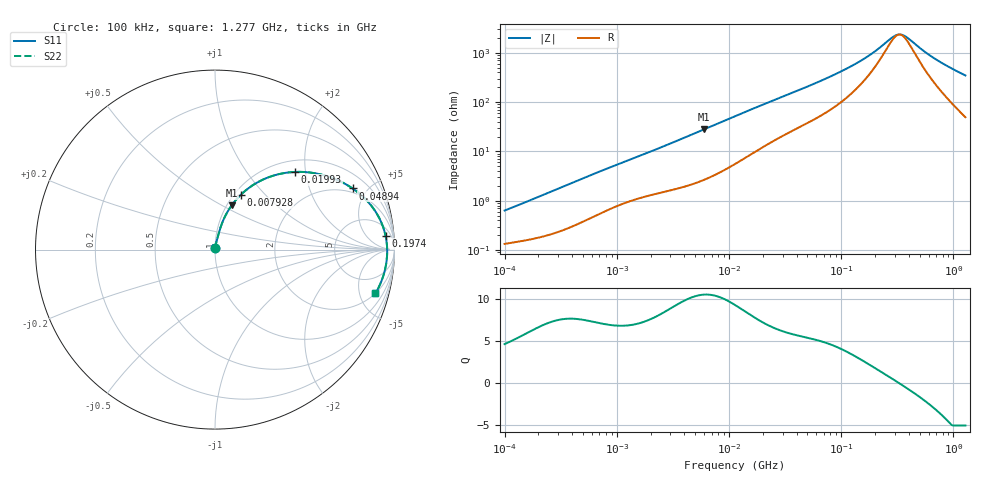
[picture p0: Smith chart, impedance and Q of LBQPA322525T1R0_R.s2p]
! LBQPA322525T1R0_R  S-PARAMETER MODEL  ( General Type )
! Model Generated by TAIYO YUDEN Corporation (http://www.ty-top.com)
! Version 1.0
! TAIYO YUDEN Control No. 191025NI43SB-FBB
! Copyright(c) 2019 TAIYO YUDEN CO.,LTD. All Rights Reserved.
! Product Description (link to TY-COMPAS)
! https://ds.yuden.co.jp/TYCOMPAS/or/detail?pn=LBQPA322525T1R0MR&u=M
! Products Name : Inductors
! Characteristics :
!  Inductance : 1.0 uH , SRF(min) : 250 MHz , DC Resistance(max) : 0.0715 Ohm
!  Rated Current : Saturation :2000 mA , Temp Rise : 1100 mA (20 degC)
!  Case Size : 3.2 x 2.5 / 0.126 x 0.098 [mm/inch] , Thickness : 2.5 / 0.098 [mm/inch]
!  (Conditions: Temperature = 25 degC , DC Bias Current/Voltage = 0A / 0V)
! External Node Assignments :
!  1  o---GGG---o  2
! GND o---------o GND
! Frequency Range : 0.1MHz  -  1277.432519MHz  [ 402 STEP ]
# MHz S RI R 50
! Freq[MHz].  S11 Real  S11 Imag  S21 Real  S21 Imag  S12 Real  S12 Imag  S22 Real  S22 Imag
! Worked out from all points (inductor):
!   401 points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, 100 kHz to 1.277 GHz, reference 50 ohm
!   read as one part in series: L = 967 nH near 104.8 kHz
!   highest Q = 10.5 at 5.97 MHz (marker M1), where L = 743 nH
!   self-resonance near 329.6 MHz
!   S11 on the Smith chart (normalised r, x): 100 kHz: 1.00, +0.01; 7.928 MHz: 1.07, +0.73; 19.93 MHz: 1.24, +1.76; 48.94 MHz: 1.74, +3.99; 197.4 MHz: 11, +18; 1.277 GHz: 1.99, -6.88
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0.1  0.00137 0.00618  0.9986 -0.00618  0.9986 -0.00618  0.00137 0.00618
0.487317  0.00441 0.0275  0.9956 -0.0275  0.9956 -0.0275  0.00441 0.0275
1.196503  0.0128 0.061  0.9872 -0.061  0.9872 -0.061  0.0128 0.061
2.374779  0.0267 0.1109  0.9733 -0.1109  0.9733 -0.1109  0.0267 0.1109
5.970231  0.0927 0.2464  0.9073 -0.2464  0.9073 -0.2464  0.0927 0.2464
7.928323  0.1421 0.304  0.8579 -0.304  0.8579 -0.304  0.1421 0.304
11.5727  0.243 0.378  0.757 -0.378  0.757 -0.378  0.243 0.378
19.93193  0.4473 0.4328  0.5527 -0.4328  0.5527 -0.4328  0.4473 0.4328
29.78987  0.6053 0.4147  0.3947 -0.4147  0.3947 -0.4147  0.6053 0.4147
48.93858  0.7663 0.341  0.2337 -0.341  0.2337 -0.341  0.7663 0.341
55.07831  0.7969 0.3184  0.2031 -0.3184  0.2031 -0.3184  0.7969 0.3184
78.51783  0.8695 0.2462  0.1305 -0.2462  0.1305 -0.2462  0.8695 0.2462
111.9324  0.9156 0.175  0.0844 -0.175  0.0844 -0.175  0.9156 0.175
152.199  0.939 0.1189  0.061 -0.1189  0.061 -0.1189  0.939 0.1189
197.395  0.9506 0.0762  0.0494 -0.0762  0.0494 -0.0762  0.9506 0.0762
268.406  0.9576 0.0298  0.0424 -0.0298  0.0424 -0.0298  0.9576 0.0298
316.7037  0.9591 0.00576  0.0409 -0.00576  0.0409 -0.00576  0.9591 0.00576
339.9779  0.9594 -0.00448  0.0406 0.00448  0.0406 0.00448  0.9594 -0.00448
364.9625  0.9593 -0.0148  0.0407 0.0148  0.0407 0.0148  0.9593 -0.0148
674.7768  0.9473 -0.1115  0.0527 0.1115  0.0527 0.1115  0.9473 -0.1115
939.468  0.9275 -0.1752  0.0725 0.1752  0.0725 0.1752  0.9275 -0.1752
1277.433  0.8938 -0.2444  0.1062 0.2444  0.1062 0.2444  0.8938 -0.2444
